[IBIS Ver]   3.2
[File name]   xc7445a-a.ibs
[File Rev]   0.2
[Date]   Tue Oct 29 11:20:04 CST 2002
[Source]   File originated at Motorola Somerset Design Center.
|   Created by Jim Nissen.
[Notes]   This IBIS model is for the Apollo 360CBGA ceramic package.
|   The driver and receiver models are characterized up to
|   2.5V mode on the system bus.
|   The convention is xc7455a-x.ibs, where -x
|   is one of the configurations of system bus voltage
|   modes. Following is a table of the code for bus combinations:
|   IBIS model   Bus mode
|   xc7445a-a.ibs  2.5V
|   xc7445a-b.ibs  1.8V
[Disclaimer]   This information is for modeling purposes only and
|   is not guaranteed.
[Component]   Apollo
[Manufacturer]  Motorola
[Package]
|   typ   min   max
R_pkg   0.0   0.0   0.0
L_pkg   0.0   0.0   0.0
C_pkg   0.0   0.0   0.0
[Pin]   signal_name   model_name   R_pin   L_pin   C_pin
A2   SRESET_B   busio   1E-016   1E-016   1E-016
A3   CKSTP_IN_B   busio   1E-016   1E-016   1E-016
A4   TDO   busio   1E-016   1E-016   1E-016
A5   TRST_B   rcvr   1E-016   1E-016   1E-016
A7   PLL_CFG(4)   busio   1E-016   1E-016   1E-016
A8   AVDD   power   1E-016   1E-016   1E-016
A9   PMON_OUT_B   busio   1E-016   1E-016   1E-016
A10   SYSCLK   busio   1E-016   1E-016   1E-016
A11   EXT_QUAL   busio   1E-016   1E-016   1E-016
A12   TEST0   busio   1E-016   1E-016   1E-016
B1   CKSTP_OUT_B   busio   1E-016   1E-016   1E-016
B2   HIT_B   busio   1E-016   1E-016   1E-016
B3   L2_TSTCLK   rcvr   1E-016   1E-016   1E-016
B6   TEST1   busio   1E-016   1E-016   1E-016
B7   BVSEL   rcvr   1E-016   1E-016   1E-016
B8   PLL_CFG(0)   busio   1E-016   1E-016   1E-016
B9   TDI   rcvr   1E-016   1E-016   1E-016
B10   TEST2   busio   1E-016   1E-016   1E-016
B11   A(35)   busio   1E-016   1E-016   1E-016
B12   A(32)   busio   1E-016   1E-016   1E-016
C1   AP(0)   busio   1E-016   1E-016   1E-016
C4   A(33)   busio   1E-016   1E-016   1E-016
C5   TT(4)   busio   1E-016   1E-016   1E-016
C6   TCK   rcvr   1E-016   1E-016   1E-016
C7   PLL_CFG(2)   busio   1E-016   1E-016   1E-016
C8   PLL_CFG(1)   busio   1E-016   1E-016   1E-016
C9   MCP_B   busio   1E-016   1E-016   1E-016
C10   A(8)   busio   1E-016   1E-016   1E-016
C11   A(2)   busio   1E-016   1E-016   1E-016
D1   A(7)   busio   1E-016   1E-016   1E-016
D2   BR_B   busio   1E-016   1E-016   1E-016
D3   WT_B   busio   1E-016   1E-016   1E-016
D4   INT_B   busio   1E-016   1E-016   1E-016
D7   PLL_CFG(3)   busio   1E-016   1E-016   1E-016
D8   HRESET_B   busio   1E-016   1E-016   1E-016
D9   PMON_IN_B   busio   1E-016   1E-016   1E-016
D10   TEST4   busio   1E-016   1E-016   1E-016
D11   A(6)   busio   1E-016   1E-016   1E-016
D12   A(10)   busio   1E-016   1E-016   1E-016
E1   TBEN   busio   1E-016   1E-016   1E-016
E2   GBL_B   busio   1E-016   1E-016   1E-016
E3   AP(1)   busio   1E-016   1E-016   1E-016
E4   SHD0_B   busio   1E-016   1E-016   1E-016
E5   TT(0)   busio   1E-016   1E-016   1E-016
E6   TT(1)   busio   1E-016   1E-016   1E-016
E7   TSIZ(2)   busio   1E-016   1E-016   1E-016
E8   LSSD_MODE_B   rcvr   1E-016   1E-016   1E-016
E9   TT(3)   busio   1E-016   1E-016   1E-016
E10   TEST3   busio   1E-016   1E-016   1E-016
E11   A(0)   busio   1E-016   1E-016   1E-016
F1   TMS   rcvr   1E-016   1E-016   1E-016
F4   A(14)   busio   1E-016   1E-016   1E-016
F5   AP(3)   busio   1E-016   1E-016   1E-016
F6   TT(2)   busio   1E-016   1E-016   1E-016
F7   TSIZ(1)   busio   1E-016   1E-016   1E-016
F8   BMODE_B(1)   busio   1E-016   1E-016   1E-016
F9   SMI_B   busio   1E-016   1E-016   1E-016
F10   A(4)   busio   1E-016   1E-016   1E-016
F11   TBST_B   busio   1E-016   1E-016   1E-016
G1   DTI(0)   busio   1E-016   1E-016   1E-016
G2   A(9)   busio   1E-016   1E-016   1E-016
G3   A(3)   busio   1E-016   1E-016   1E-016
G4   A(12)   busio   1E-016   1E-016   1E-016
G5   QACK_B   busio   1E-016   1E-016   1E-016
G6   TSIZ(0)   busio   1E-016   1E-016   1E-016
G7   AP(4)   busio   1E-016   1E-016   1E-016
G8   L1_TSTCLK   rcvr   1E-016   1E-016   1E-016
G9   BMODE_B(0)   busio   1E-016   1E-016   1E-016
G10   A(34)   busio   1E-016   1E-016   1E-016
H1   A(1)   busio   1E-016   1E-016   1E-016
H2   CLK_OUT   busio   1E-016   1E-016   1E-016
H5   SHD1_B   busio   1E-016   1E-016   1E-016
H6   AP(2)   busio   1E-016   1E-016   1E-016
J1   CI_B   busio   1E-016   1E-016   1E-016
J2   A(20)   busio   1E-016   1E-016   1E-016
J3   A(23)   busio   1E-016   1E-016   1E-016
J4   A(16)   busio   1E-016   1E-016   1E-016
K1   DTI(1)   busio   1E-016   1E-016   1E-016
K4   A(21)   busio   1E-016   1E-016   1E-016
K5   A(18)   busio   1E-016   1E-016   1E-016
K6   TA_B   busio   1E-016   1E-016   1E-016
L1   TEA_B   busio   1E-016   1E-016   1E-016
L2   A(5)   busio   1E-016   1E-016   1E-016
L3   A(11)   busio   1E-016   1E-016   1E-016
L4   TS_B   busio   1E-016   1E-016   1E-016
M1   BG_B   busio   1E-016   1E-016   1E-016
M2   DBG_B   busio   1E-016   1E-016   1E-016
M5   A(24)   busio   1E-016   1E-016   1E-016
M6   DP(4)   busio   1E-016   1E-016   1E-016
N1   DTI(3)   busio   1E-016   1E-016   1E-016
N2   ARTRY_B   busio   1E-016   1E-016   1E-016
N3   A(26)   busio   1E-016   1E-016   1E-016
N4   A(22)   busio   1E-016   1E-016   1E-016
N5   A(30)   busio   1E-016   1E-016   1E-016
N8   DP(6)   busio   1E-016   1E-016   1E-016
N9   D(25)   busio   1E-016   1E-016   1E-016
N10   D(19)   busio   1E-016   1E-016   1E-016
N11   D(18)   busio   1E-016   1E-016   1E-016
P1   DTI(2)   busio   1E-016   1E-016   1E-016
P4   QREQ_B   busio   1E-016   1E-016   1E-016
P5   A(25)   busio   1E-016   1E-016   1E-016
P6   D(60)   busio   1E-016   1E-016   1E-016
P7   D(38)   busio   1E-016   1E-016   1E-016
P10   D(26)   busio   1E-016   1E-016   1E-016
P13   D(11)   busio   1E-016   1E-016   1E-016
P14   D(7)   busio   1E-016   1E-016   1E-016
P17   D(40)   busio   1E-016   1E-016   1E-016
R1   AACK_B   busio   1E-016   1E-016   1E-016
R2   A(17)   busio   1E-016   1E-016   1E-016
R3   DRDY_B   busio   1E-016   1E-016   1E-016
R6   D(37)   busio   1E-016   1E-016   1E-016
R7   D(59)   busio   1E-016   1E-016   1E-016
R8   D(61)   busio   1E-016   1E-016   1E-016
R9   D(28)   busio   1E-016   1E-016   1E-016
R10   D(24)   busio   1E-016   1E-016   1E-016
R11   D(20)   busio   1E-016   1E-016   1E-016
R12   D(14)   busio   1E-016   1E-016   1E-016
R15   D(0)   busio   1E-016   1E-016   1E-016
R18   D(43)   busio   1E-016   1E-016   1E-016
R19   D(41)   busio   1E-016   1E-016   1E-016
T1   A(27)   busio   1E-016   1E-016   1E-016
T2   A(13)   busio   1E-016   1E-016   1E-016
T3   DP(0)   busio   1E-016   1E-016   1E-016
T4   DP(2)   busio   1E-016   1E-016   1E-016
T5   D(34)   busio   1E-016   1E-016   1E-016
T8   D(63)   busio   1E-016   1E-016   1E-016
T11   D(23)   busio   1E-016   1E-016   1E-016
T12   D(15)   busio   1E-016   1E-016   1E-016
T13   D(10)   busio   1E-016   1E-016   1E-016
T14   D(2)   busio   1E-016   1E-016   1E-016
T15   D(5)   busio   1E-016   1E-016   1E-016
T16   D(51)   busio   1E-016   1E-016   1E-016
T17   D(53)   busio   1E-016   1E-016   1E-016
T18   D(52)   busio   1E-016   1E-016   1E-016
T19   D(45)   busio   1E-016   1E-016   1E-016
U1   A(29)   busio   1E-016   1E-016   1E-016
U4   D(56)   busio   1E-016   1E-016   1E-016
U5   D(35)   busio   1E-016   1E-016   1E-016
U6   D(33)   busio   1E-016   1E-016   1E-016
U7   D(58)   busio   1E-016   1E-016   1E-016
U8   D(57)   busio   1E-016   1E-016   1E-016
U9   D(30)   busio   1E-016   1E-016   1E-016
U10   D(27)   busio   1E-016   1E-016   1E-016
U11   D(21)   busio   1E-016   1E-016   1E-016
U14   D(12)   busio   1E-016   1E-016   1E-016
U15   D(6)   busio   1E-016   1E-016   1E-016
U18   D(48)   busio   1E-016   1E-016   1E-016
U19   D(46)   busio   1E-016   1E-016   1E-016
V1   A(15)   busio   1E-016   1E-016   1E-016
V2   A(28)   busio   1E-016   1E-016   1E-016
V3   DP(5)   busio   1E-016   1E-016   1E-016
V6   D(39)   busio   1E-016   1E-016   1E-016
V9   D(31)   busio   1E-016   1E-016   1E-016
V12   D(17)   busio   1E-016   1E-016   1E-016
V13   D(8)   busio   1E-016   1E-016   1E-016
V16   D(3)   busio   1E-016   1E-016   1E-016
V17   D(55)   busio   1E-016   1E-016   1E-016
V18   D(42)   busio   1E-016   1E-016   1E-016
V19   D(44)   busio   1E-016   1E-016   1E-016
W1   A(31)   busio   1E-016   1E-016   1E-016
W2   A(19)   busio   1E-016   1E-016   1E-016
W3   D(54)   busio   1E-016   1E-016   1E-016
W4   DP(1)   busio   1E-016   1E-016   1E-016
W5   D(32)   busio   1E-016   1E-016   1E-016
W6   DP(7)   busio   1E-016   1E-016   1E-016
W7   D(36)   busio   1E-016   1E-016   1E-016
W8   D(62)   busio   1E-016   1E-016   1E-016
W9   DP(3)   busio   1E-016   1E-016   1E-016
W10   D(29)   busio   1E-016   1E-016   1E-016
W11   D(22)   busio   1E-016   1E-016   1E-016
W12   D(16)   busio   1E-016   1E-016   1E-016
W13   D(9)   busio   1E-016   1E-016   1E-016
W14   D(13)   busio   1E-016   1E-016   1E-016
W15   D(1)   busio   1E-016   1E-016   1E-016
W16   D(4)   busio   1E-016   1E-016   1E-016
W17   D(49)   busio   1E-016   1E-016   1E-016
W18   D(50)   busio   1E-016   1E-016   1E-016
W19   D(47)   busio   1E-016   1E-016   1E-016
|!!!![Package Model] 'name'  calls name
[Package Model] apollo_360
[Define Package Model] apollo_360
[Manufacturer] Motorola Inc.
[OEM] Motorola Inc.
[Description] Apollo 6 360 CBGA Package T-Line pkg model
[Number Of Sections] 23
[Number Of Pins]  178
[Pin Numbers]
|Although any length unit can be used for Len, mm is used here.
|signal (1)SYSCLK
A10   Len=0 L=0.01n /
Len=9.505981 L=0.457002655n C=0.272728196p R=0.0080 /
Len=0 L=0.01n /
Len=0 L=0.01n /
Len=0 L=0.01n /
Len=0 L=0.01n /
Len=0 L=0.01n /
Len=0 L=0.027n /
|signal (2)EXT_QUAL
A11   Len=0 L=0.01n /
Len=8.151963 L=0.457002655n C=0.272728196p R=0.0080 /
Len=0 L=0.01n /
Len=0 L=0.01n /
Len=0 L=0.01n /
Len=0 L=0.01n /
Len=0 L=0.01n /
Len=0 L=0.027n /
|signal (3)TEST0 (CHKS_)
A12   Len=0 L=0.01n /
Len=8.249788 L=0.457002655n C=0.272728196p R=0.0080 /
Len=0 L=0.01n /
Len=0 L=0.01n /
Len=0 L=0.01n /
Len=0 L=0.01n /
Len=0 L=0.01n /
Len=0 L=0.027n /
|signal (11)SRESET_
A2   Len=0 L=0.01n /
Len=11.989745 L=0.457002655n C=0.272728196p R=0.0080 /
Len=0 L=0.01n /
Len=0 L=0.01n /
Len=0 L=0.01n /
Len=0 L=0.01n /
Len=0 L=0.01n /
Len=0 L=0.027n /
|signal (12)CKSTP_IN_
A3   Len=0 L=0.01n /
Len=0 L=0.01n /
Len=0 L=0.01n /
Len=11.447296 L=0.381951499n C=0.27016304p R=0.008101266 /
Len=0 L=0.01n /
Len=0 L=0.01n /
Len=0 L=0.01n /
Len=0 L=0.027n /
|signal (13)TDO
A4   Len=0 L=0.01n /
Len=10.401228 L=0.457388623n C=0.23790985p R=0.008205128 /
Len=0 L=0.01n /
Len=0 L=0.01n /
Len=0 L=0.01n /
Len=0 L=0.01n /
Len=0 L=0.01n /
Len=0 L=0.027n /
|signal (14)TRST_
A5   Len=0 L=0.01n /
Len=8.331435 L=0.457259141n C=0.23935889p R=0.008135593 /
Len=0 L=0.01n /
Len=0 L=0.01n /
Len=0 L=0.01n /
Len=0 L=0.01n /
Len=0 L=0.01n /
Len=0 L=0.027n /
|signal (16)PLL_CFG4
A7   Len=0 L=0.01n /
Len=0 L=0.01n /
Len=0 L=0.01n /
Len=8.255493 L=0.3797849542n C=0.297875648p R=0.0080 /
Len=0 L=0.01n /
Len=0 L=0.01n /
Len=0 L=0.01n /
Len=0 L=0.027n /
|signal (17)AVDD
A8   Len=0 L=0.01n /
Len=0 L=0.01n /
Len=0 L=0.01n /
Len=0 L=0.01n /
Len=0 L=0.01n /
Len=8.095418 L=0.11320642n C=0.4661983p R=0.0043076924 /
Len=0 L=0.01n /
Len=0 L=0.027n /
|signal (18)PMON_OUT_
A9   Len=0 L=0.01n /
Len=7.4271607 L=0.457002655n C=0.272728196p R=0.0080 /
Len=0 L=0.01n /
Len=0 L=0.01n /
Len=0 L=0.01n /
Len=0 L=0.01n /
Len=0 L=0.01n /
Len=0 L=0.027n /
|signal (19)CKSTP_OUT_
B1   Len=0 L=0.01n /
Len=0 L=0.01n /
Len=0 L=0.01n /
Len=13.635491 L=0.3819750673n C=0.3588282p R=0.008247423 /
Len=0 L=0.01n /
Len=0 L=0.01n /
Len=0 L=0.01n /
Len=0 L=0.027n /
|signal (20)TEST2 (SRW0)
B10   Len=0 L=0.01n /
Len=0 L=0.01n /
Len=0 L=0.01n /
Len=6.3558884 L=0.3797849542n C=0.297875648p R=0.0080 /
Len=0 L=0.01n /
Len=0 L=0.01n /
Len=0 L=0.01n /
Len=0 L=0.027n /
|signal (21)A35
B11   Len=0 L=0.01n /
Len=6.712278 L=0.457002655n C=0.272728196p R=0.0080 /
Len=0 L=0.01n /
Len=0 L=0.01n /
Len=0 L=0.01n /
Len=0 L=0.01n /
Len=0 L=0.01n /
Len=0 L=0.027n /
|signal (22)A32
B12   Len=0 L=0.01n /
Len=0 L=0.01n /
Len=0 L=0.01n /
Len=7.6983905 L=0.3797849542n C=0.297875648p R=0.0080 /
Len=0 L=0.01n /
Len=0 L=0.01n /
Len=0 L=0.01n /
Len=0 L=0.027n /
|signal (30)HIT_
B2   Len=0 L=0.01n /
Len=0 L=0.01n /
Len=0 L=0.01n /
Len=11.587751 L=0.3819682849n C=0.36109874p R=0.008205128 /
Len=0 L=0.01n /
Len=0 L=0.01n /
Len=0 L=0.01n /
Len=0 L=0.027n /
|signal (31)L2_TSTCLK
B3   Len=0 L=0.01n /
Len=0 L=0.01n /
Len=0 L=0.01n /
Len=0 L=0.01n /
Len=0 L=0.01n /
Len=9.688901 L=0.457783149n C=0.272728196p R=0.0080 /
Len=0 L=0.01n /
Len=0 L=0.027n /
|signal (32)TEST1 (IARTRY0_)
B6   Len=0 L=0.01n /
Len=0 L=0.01n /
Len=0 L=0.01n /
Len=7.2262797 L=0.3797849542n C=0.297875648p R=0.0080 /
Len=0 L=0.01n /
Len=0 L=0.01n /
Len=0 L=0.01n /
Len=0 L=0.027n /
|signal (33)BVSEL
B7   Len=0 L=0.01n /
Len=0 L=0.01n /
Len=0 L=0.01n /
Len=6.886 L=0.3797849542n C=0.297875648p R=0.0080 /
Len=0 L=0.01n /
Len=0 L=0.01n /
Len=0 L=0.01n /
Len=0 L=0.027n /
|signal (34)PLL_CFG0
B8   Len=0 L=0.01n /
Len=6.5972886 L=0.457002655n C=0.272728196p R=0.0080 /
Len=0 L=0.01n /
Len=0 L=0.01n /
Len=1.0557107 L=0.3797849542n C=0.297875648p R=0.0080 /
Len=0 L=0.01n /
Len=0 L=0.01n /
Len=0 L=0.01n /
Len=0 L=0.027n /
|signal (35)TDI
B9   Len=0 L=0.01n /
Len=6.0833716 L=0.457002655n C=0.272728196p R=0.0080 /
Len=0 L=0.01n /
Len=0 L=0.01n /
Len=0 L=0.01n /
Len=0 L=0.01n /
Len=0 L=0.01n /
Len=0 L=0.027n /
|signal (36)AP0
C1   Len=0 L=0.01n /
Len=10.373757 L=0.457130489n C=0.24081622p R=0.008067227 /
Len=0 L=0.01n /
Len=0 L=0.01n /
Len=0 L=0.01n /
Len=0 L=0.01n /
Len=0 L=0.01n /
Len=0 L=0.027n /
|signal (37)A8
C10   Len=0 L=0.01n /
Len=0 L=0.01n /
Len=0 L=0.01n /
Len=0 L=0.01n /
Len=0 L=0.01n /
Len=5.8139324 L=0.457783149n C=0.272728196p R=0.0080 /
Len=0 L=0.01n /
Len=0 L=0.027n /
|signal (38)A2
C11   Len=0 L=0.01n /
Len=0 L=0.01n /
Len=0 L=0.01n /
Len=0 L=0.01n /
Len=0 L=0.01n /
Len=7.043373 L=0.457783149n C=0.272728196p R=0.0080 /
Len=0 L=0.01n /
Len=0 L=0.027n /
|signal (46)A33
C4   Len=0 L=0.01n /
Len=7.562751 L=0.457259141n C=0.23935889p R=0.008135593 /
Len=0 L=0.01n /
Len=0 L=0.01n /
Len=0 L=0.01n /
Len=0 L=0.01n /
Len=0 L=0.01n /
Len=0 L=0.027n /
|signal (47)TT4
C5   Len=0 L=0.01n /
Len=7.937086 L=0.457388623n C=0.23790985p R=0.008205128 /
Len=0 L=0.01n /
Len=0 L=0.01n /
Len=0 L=0.01n /
Len=0 L=0.01n /
Len=0 L=0.01n /
Len=0 L=0.027n /
|signal (48)TCK
C6   Len=0 L=0.01n /
Len=0 L=0.01n /
Len=0 L=0.01n /
Len=6.6086226 L=0.3797849542n C=0.297875648p R=0.0080 /
Len=0 L=0.01n /
Len=0 L=0.01n /
Len=0 L=0.01n /
Len=0 L=0.027n /
|signal (49)PLL_CFG2
C7   Len=0 L=0.01n /
Len=4.6758094 L=0.457002655n C=0.272728196p R=0.0080 /
Len=0 L=0.01n /
Len=0 L=0.01n /
Len=2.2450335 L=0.3797849542n C=0.297875648p R=0.0080 /
Len=0 L=0.01n /
Len=0 L=0.01n /
Len=0 L=0.01n /
Len=0 L=0.027n /
|signal (50)PLL_CFG1
C8   Len=0 L=0.01n /
Len=3.603795 L=0.457002655n C=0.272728196p R=0.0080 /
Len=0 L=0.01n /
Len=0 L=0.01n /
Len=0 L=0.01n /
Len=0 L=0.01n /
Len=4.5483403 L=0.457783149n C=0.272728196p R=0.0080 /
Len=0 L=0.01n /
Len=0 L=0.027n /
|signal (51)MCP_
C9   Len=0 L=0.01n /
Len=0 L=0.01n /
Len=0 L=0.01n /
Len=5.0013967 L=0.3797849542n C=0.297875648p R=0.0080 /
Len=0 L=0.01n /
Len=0 L=0.01n /
Len=0 L=0.01n /
Len=0 L=0.027n /
|signal (52)A7
D1   Len=0 L=0.01n /
Len=9.550656 L=0.457259141n C=0.23935889p R=0.008135593 /
Len=0 L=0.01n /
Len=0 L=0.01n /
Len=0 L=0.01n /
Len=0 L=0.01n /
Len=0 L=0.01n /
Len=0 L=0.027n /
|signal (53)TEST4 (DX_)
D10   Len=0 L=0.01n /
Len=3.5534408 L=0.457002655n C=0.272728196p R=0.0080 /
Len=0 L=0.01n /
Len=0 L=0.01n /
Len=0 L=0.01n /
Len=0 L=0.01n /
Len=0 L=0.01n /
Len=0 L=0.027n /
|signal (54)A6
D11   Len=0 L=0.01n /
Len=0 L=0.01n /
Len=0 L=0.01n /
Len=4.709767 L=0.3819682849n C=0.36109874p R=0.008205128 /
Len=0 L=0.01n /
Len=0 L=0.01n /
Len=1.7698662 L=0.457783149n C=0.272728196p R=0.0080 /
Len=0 L=0.01n /
Len=0 L=0.027n /
|signal (55)A10
D12   Len=0 L=0.01n /
Len=6.0452266 L=0.457002655n C=0.272728196p R=0.0080 /
Len=0 L=0.01n /
Len=0 L=0.01n /
Len=0 L=0.01n /
Len=0 L=0.01n /
Len=1.2421368 L=0.457783149n C=0.272728196p R=0.0080 /
Len=0 L=0.01n /
Len=0 L=0.027n /
|signal (62)BR_
D2   Len=0 L=0.01n /
Len=8.308557 L=0.457194711n C=0.24008651p R=0.008101266 /
Len=0 L=0.01n /
Len=0 L=0.01n /
Len=0 L=0.01n /
Len=0 L=0.01n /
Len=0 L=0.01n /
Len=0 L=0.027n /
|signal (63)WT_
D3   Len=0 L=0.01n /
Len=0 L=0.01n /
Len=0 L=0.01n /
Len=8.110517 L=0.3819750673n C=0.3588282p R=0.008247423 /
Len=0 L=0.01n /
Len=0 L=0.01n /
Len=0 L=0.01n /
Len=0 L=0.027n /
|signal (64)INT_
D4   Len=0 L=0.01n /
Len=5.376824 L=0.457388623n C=0.23790985p R=0.008205128 /
Len=0 L=0.01n /
Len=0 L=0.01n /
Len=0 L=0.01n /
Len=0 L=0.01n /
Len=0 L=0.01n /
Len=0 L=0.027n /
|signal (65)PLL_CFG3
D7   Len=0 L=0.01n /
Len=4.341307 L=0.457002655n C=0.272728196p R=0.0080 /
Len=0 L=0.01n /
Len=0 L=0.01n /
Len=0 L=0.01n /
Len=0 L=0.01n /
Len=0 L=0.01n /
Len=0 L=0.027n /
|signal (66)HRESET_
D8   Len=0 L=0.01n /
Len=2.9926438 L=0.457002655n C=0.272728196p R=0.0080 /
Len=0 L=0.01n /
Len=0 L=0.01n /
Len=0 L=0.01n /
Len=0 L=0.01n /
Len=2.6308246 L=0.457783149n C=0.272728196p R=0.0080 /
Len=0 L=0.01n /
Len=0 L=0.027n /
|signal (67)PMON_IN_
D9   Len=0 L=0.01n /
Len=3.392897 L=0.457002655n C=0.272728196p R=0.0080 /
Len=0 L=0.01n /
Len=0 L=0.01n /
Len=0 L=0.01n /
Len=0 L=0.01n /
Len=0 L=0.01n /
Len=0 L=0.027n /
|signal (68)TBEN
E1   Len=0 L=0.01n /
Len=7.6689763 L=0.457388623n C=0.23790985p R=0.008205128 /
Len=0 L=0.01n /
Len=0 L=0.01n /
Len=0 L=0.01n /
Len=0 L=0.01n /
Len=0 L=0.01n /
Len=0 L=0.027n /
|signal (69)TEST3 (SRW1_)
E10   Len=0 L=0.01n /
Len=0 L=0.01n /
Len=0 L=0.01n /
Len=0 L=0.01n /
Len=0 L=0.01n /
Len=3.1916661 L=0.457783149n C=0.272728196p R=0.0080 /
Len=0 L=0.01n /
Len=0 L=0.027n /
|signal (70)A0
E11   Len=0 L=0.01n /
Len=0 L=0.01n /
Len=0 L=0.01n /
Len=2.1588755 L=0.3927025875n C=0.34993997p R=0.008421052 /
Len=0 L=0.01n /
Len=0 L=0.01n /
Len=1.7472317 L=0.457783149n C=0.272728196p R=0.0080 /
Len=0 L=0.01n /
Len=0 L=0.027n /
|signal (77)GBL_
E2   Len=0 L=0.01n /
Len=0 L=0.01n /
Len=0 L=0.01n /
Len=8.544575 L=0.3819750673n C=0.3588282p R=0.008247423 /
Len=0 L=0.01n /
Len=0 L=0.01n /
Len=0 L=0.01n /
Len=0 L=0.027n /
|signal (78)AP1
E3   Len=0 L=0.01n /
Len=6.469437 L=0.457259141n C=0.23935889p R=0.008135593 /
Len=0 L=0.01n /
Len=0 L=0.01n /
Len=0 L=0.01n /
Len=0 L=0.01n /
Len=0 L=0.01n /
Len=0 L=0.027n /
|signal (79)SHD0_
E4   Len=0 L=0.01n /
Len=0 L=0.01n /
Len=0 L=0.01n /
Len=5.9466734 L=0.3819853138n C=0.35545915p R=0.008311688 /
Len=0 L=0.01n /
Len=0 L=0.01n /
Len=0 L=0.01n /
Len=0 L=0.027n /
|signal (80)TT0
E5   Len=0 L=0.01n /
Len=3.4525087 L=0.457782161n C=0.23361155p R=0.008421052 /
Len=0 L=0.01n /
Len=0 L=0.01n /
Len=0 L=0.01n /
Len=0 L=0.01n /
Len=0 L=0.01n /
Len=0 L=0.027n /
|signal (81)TT1
E6   Len=0 L=0.01n /
Len=2.3488173 L=0.457002655n C=0.272728196p R=0.0080 /
Len=0 L=0.01n /
Len=0 L=0.01n /
Len=0 L=0.01n /
Len=0 L=0.01n /
Len=0 L=0.01n /
Len=0 L=0.027n /
|signal (82)TSIZ2
E7   Len=0 L=0.01n /
Len=3.767044 L=0.4572223n C=0.2397744p R=0.008115943 /
Len=0 L=0.01n /
Len=0 L=0.01n /
Len=0 L=0.01n /
Len=0 L=0.01n /
Len=0 L=0.01n /
Len=0 L=0.027n /
|signal (83)LSSD_MODE_
E8   Len=0 L=0.01n /
Len=0 L=0.01n /
Len=0 L=0.01n /
Len=2.857981 L=0.3819731254n C=0.35947493p R=0.008235293 /
Len=0 L=0.01n /
Len=0 L=0.01n /
Len=0 L=0.01n /
Len=0 L=0.027n /
|signal (84)TT3
E9   Len=0 L=0.01n /
Len=2.1635232 L=0.457002655n C=0.272728196p R=0.0080 /
Len=0 L=0.01n /
Len=0 L=0.01n /
Len=0 L=0.01n /
Len=0 L=0.01n /
Len=0 L=0.01n /
Len=0 L=0.027n /
|signal (85)TMS
F1   Len=0 L=0.01n /
Len=4.6419873 L=0.457782161n C=0.23361155p R=0.008421052 /
Len=0 L=0.01n /
Len=0 L=0.01n /
Len=3.5738835 L=0.3797849542n C=0.297875648p R=0.0080 /
Len=0 L=0.01n /
Len=0 L=0.01n /
Len=0 L=0.01n /
Len=0 L=0.027n /
|signal (86)A4
F10   Len=0 L=0.01n /
Len=0 L=0.01n /
Len=0 L=0.01n /
Len=0 L=0.01n /
Len=0 L=0.01n /
Len=1.6332662 L=0.457783149n C=0.272728196p R=0.0080 /
Len=0 L=0.01n /
Len=0 L=0.027n /
|signal (87)TBST_
F11   Len=0 L=0.01n /
Len=0 L=0.01n /
Len=0 L=0.01n /
Len=0 L=0.01n /
Len=0 L=0.01n /
Len=2.1101484 L=0.457783149n C=0.272728196p R=0.0080 /
Len=0 L=0.01n /
Len=0 L=0.027n /
|signal (96)A14
F4   Len=0 L=0.01n /
Len=0 L=0.01n /
Len=0 L=0.01n /
Len=0 L=0.01n /
Len=0 L=0.01n /
Len=5.05428 L=0.457783149n C=0.272728196p R=0.0080 /
Len=0 L=0.01n /
Len=0 L=0.027n /
|signal (97)AP3
F5   Len=0 L=0.01n /
Len=0 L=0.01n /
Len=0 L=0.01n /
Len=2.191985 L=0.3797849542n C=0.297875648p R=0.0080 /
Len=0 L=0.01n /
Len=0 L=0.01n /
Len=1.11173 L=0.392743277n C=0.22522578p R=0.008888889 /
Len=0 L=0.01n /
Len=0 L=0.027n /
|signal (98)TT2
F6   Len=0 L=0.01n /
Len=0 L=0.01n /
Len=0 L=0.01n /
Len=3.1034834 L=0.3819615415n C=0.36338925p R=0.008163265 /
Len=0 L=0.01n /
Len=0 L=0.01n /
Len=0 L=0.01n /
Len=0 L=0.027n /
|signal (99)TSIZ1
F7   Len=0 L=0.01n /
Len=0 L=0.01n /
Len=0 L=0.01n /
Len=2.2707162 L=0.3797849542n C=0.297875648p R=0.0080 /
Len=0 L=0.01n /
Len=0 L=0.01n /
Len=0 L=0.01n /
Len=0 L=0.027n /
|signal (100)BMODE1_
F8   Len=0 L=0.01n /
Len=1.0703574 L=0.457002655n C=0.272728196p R=0.0080 /
Len=0 L=0.01n /
Len=0 L=0.01n /
Len=0 L=0.01n /
Len=0 L=0.01n /
Len=0 L=0.01n /
Len=0 L=0.027n /
|signal (101)SMI_
F9   Len=0 L=0.01n /
Len=0 L=0.01n /
Len=0 L=0.01n /
Len=1.1542448 L=0.3797849542n C=0.297875648p R=0.0080 /
Len=0 L=0.01n /
Len=0 L=0.01n /
Len=0 L=0.01n /
Len=0 L=0.027n /
|signal (102)DTI0
G1   Len=0 L=0.01n /
Len=6.9930954 L=0.457259141n C=0.23935889p R=0.008135593 /
Len=0 L=0.01n /
Len=0 L=0.01n /
Len=0 L=0.01n /
Len=0 L=0.01n /
Len=0 L=0.01n /
Len=0 L=0.027n /
|signal (103)A34
G10   Len=0 L=0.01n /
Len=0 L=0.01n /
Len=0 L=0.01n /
Len=0 L=0.01n /
Len=0 L=0.01n /
Len=0.5990488 L=0.457783149n C=0.272728196p R=0.0080 /
Len=0 L=0.01n /
Len=0 L=0.027n /
|signal (111)A9
G2   Len=0 L=0.01n /
Len=5.256943 L=0.457518947n C=0.23646902p R=0.008275862 /
Len=0 L=0.01n /
Len=0 L=0.01n /
Len=0 L=0.01n /
Len=0 L=0.01n /
Len=0 L=0.01n /
Len=0 L=0.027n /
|signal (112)A3
G3   Len=0 L=0.01n /
Len=0 L=0.01n /
Len=0 L=0.01n /
Len=4.7154436 L=0.3819615415n C=0.36338925p R=0.008163265 /
Len=0 L=0.01n /
Len=0 L=0.01n /
Len=0 L=0.01n /
Len=0 L=0.027n /
|signal (113)A12
G4   Len=0 L=0.01n /
Len=0 L=0.01n /
Len=0 L=0.01n /
Len=6.881833 L=0.381951499n C=0.27016304p R=0.008101266 /
Len=0 L=0.01n /
Len=0 L=0.01n /
Len=0 L=0.01n /
Len=0 L=0.027n /
|signal (114)QACK_
G5   Len=0 L=0.01n /
Len=0 L=0.01n /
Len=0 L=0.01n /
Len=0 L=0.01n /
Len=0 L=0.01n /
Len=2.4373822 L=0.457783149n C=0.272728196p R=0.0080 /
Len=0 L=0.01n /
Len=0 L=0.027n /
|signal (115)TSIZ0
G6   Len=0 L=0.01n /
Len=0 L=0.01n /
Len=0 L=0.01n /
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[End Package Model]
| Models and submodels in the file (2): busio (I/O), rcvr (Input)
